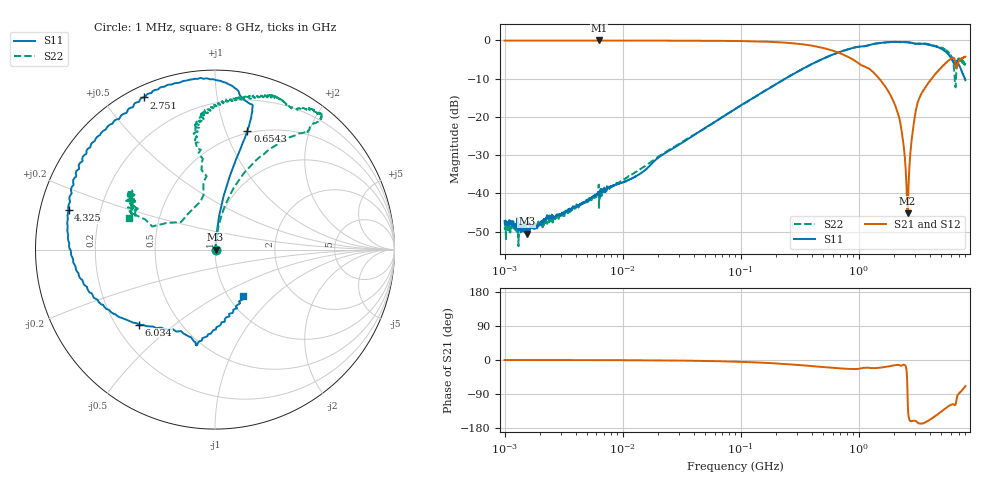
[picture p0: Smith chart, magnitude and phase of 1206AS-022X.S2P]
!s-Parameter Generated by FASTRON Sdn. Bhd.
!FASTRON P/N : 1206AS-022X
!Keysight Technologies: E5071C_MY46733604_B.14.02
!Date: Wed Nov 15 09:47:32 2023
!Version  :Rev00  Wed Nov 15 09:47:32 2023
!Data & Calibration Information:
!Freq  S11:SOLT2(ON)  S21:SOLT2(ON)  S12:SOLT2(ON)  S22:SOLT2(ON)
!PortZ  Port1:50+j0  Port2:50+j0
!When reading reference impedance value at option line is always used.
! Remarks : This data is being provided solely for informational purposes.
# Hz S dB R 50
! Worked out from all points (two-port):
!   1601 points, 1 MHz to 8 GHz, reference 50 ohm
!   highest |S21| = 0.01 dB at 6.301 MHz (marker M1); lowest = -45.2 dB at 2.59 GHz (marker M2)
!   |S21| within 3 dB of the highest: start of sweep to 646.2 MHz
!   lowest |S11| = -50.5 dB at 1.541 MHz (marker M3), VSWR 1.01, Z = 50.3 + j0.028 ohm
!   |S11| at or under -10 dB: start of sweep to 238 MHz; 7.93 GHz to end of sweep
!   |S22| runs from -53.8 to -0.4 dB; largest |S21 - S12| = 0.0068
!   S11 on the Smith chart (normalised r, x): 1 MHz: 1.01, -0.00; 654.3 MHz: 0.47, +1.19; 2.751 GHz: 0.05, +0.63; 4.325 GHz: 0.09, +0.13; 6.034 GHz: 0.29, -0.38; 8 GHz: 1.16, -0.66
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1000000  -47.19 -12.0  -0.03 -0.2  -0.04 -0.1  -48.86 -12.3
1541011  -50.51 5.3  -0.03 -0.2  -0.03 -0.2  -47.91 -10.6
4479405  -42.52 58.2  -0.04 -0.3  -0.04 -0.3  -42.94 63.0
6301378  -39.59 52.3  0.01 -0.3  -0.05 -0.4  -44.04 61.3
2.00676e7  -30.62 80.3  -0.04 -1.1  -0.06 -1.0  -30.39 79.3
8.994653e7  -17.87 83.6  -0.13 -4.4  -0.14 -4.3  -17.93 81.4
4.006501e8  -6.17 77.2  -1.36 -16.1  -1.37 -16.1  -6.18 67.7
6.54293e8  -3.25 74.7  -3.05 -21.7  -3.06 -21.8  -3.26 59.2
1.041574e9  -1.57 75.8  -6.41 -22.1  -6.41 -22.1  -1.62 51.4
1.7949e9  -0.46 91.5  -13.51 -16.9  -13.53 -17.1  -0.45 51.4
2.189041e9  -0.39 100.6  -19.92 -13.1  -19.95 -13.4  -0.42 53.1
2.589603e9  -0.45 111.2  -45.19 -93.2  -45.23 -93.3  -0.48 56.5
2.662964e9  -0.50 112.8  -35.08 -153.9  -35.13 -154.1  -0.53 56.6
2.750998e9  -0.57 115.1  -28.62 -161.5  -28.65 -161.6  -0.62 57.0
2.927065e9  -0.76 120.2  -21.59 -160.3  -21.62 -160.4  -0.85 59.5
3.162936e9  -0.83 128.5  -16.14 -165.7  -16.17 -165.8  -0.89 63.8
4.324643e9  -1.46 164.9  -9.27 -150.2  -9.26 -150.3  -1.31 81.1
5.136407e9  -2.38 -167.3  -6.73 -133.0  -6.69 -133.2  -1.99 92.1
6.033702e9  -4.51 -135.4  -4.78 -118.3  -4.77 -118.6  -3.86 99.2
6.689135e9  -5.35 -101.5  -7.16 -109.6  -7.14 -110.0  -8.57 159.8
7.074683e9  -6.50 -94.6  -5.31 -87.8  -5.30 -88.3  -4.66 146.7
8e9  -10.41 -59.2  -4.25 -68.6  -4.24 -69.1  -5.86 159.9
